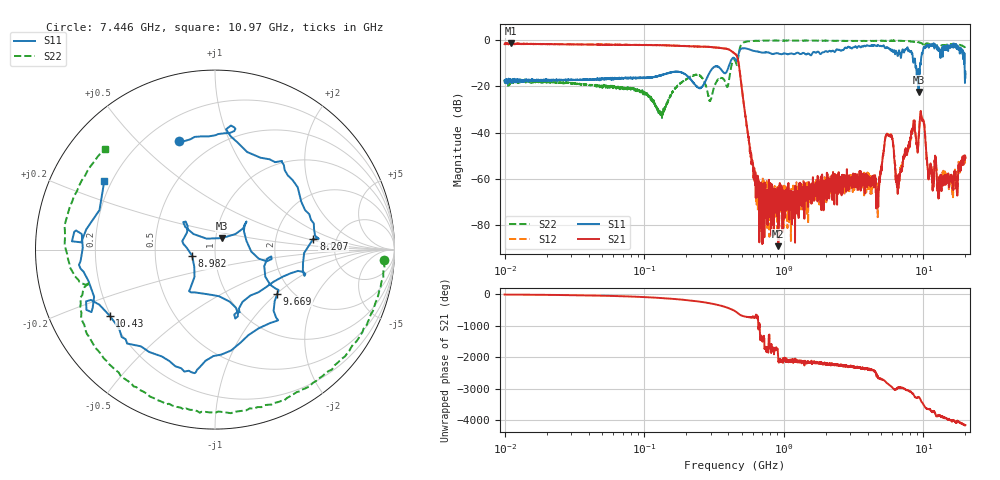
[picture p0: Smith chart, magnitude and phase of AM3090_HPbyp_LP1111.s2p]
# Hz S DB R 50
!freq MagS11 AngS11 MagS21 AngS21 MagS12 AngS12 MagS22 AngS22
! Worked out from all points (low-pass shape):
!   3201 points, 10 MHz to 20 GHz, reference 50 ohm
!   highest |S21| = -1.43 dB at 11.1 MHz (marker M1); lowest = -88.9 dB at 914.2 MHz (marker M2)
!   |S21| within 3 dB of the highest: start of sweep to 413 MHz
!   lowest |S11| = -22.5 dB at 9.242 GHz (marker M3), VSWR 1.16, Z = 53.7 + j6.91 ohm
!   |S11| at or under -10 dB: start of sweep to 410.8 MHz; 8.743 GHz to 9.483 GHz (740 MHz wide, 8.12 % of centre); 19.73 GHz to end of sweep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
!   |S22| runs from -33.7 to -0.2 dB; largest |S21 - S12| = 0.046
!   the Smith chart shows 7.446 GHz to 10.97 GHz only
!   S11 on the Smith chart (normalised r, x): 7.446 GHz: 0.33, +0.67; 8.207 GHz: 3.35, +0.59; 8.982 GHz: 0.77, -0.06; 9.669 GHz: 1.68, -1.01; 10.43 GHz: 0.20, -0.28; 10.97 GHz: 0.17, +0.28
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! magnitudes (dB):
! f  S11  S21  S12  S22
! 10 MHz  -17.5  -1.8  -1.5  -17.7
! 11.1 MHz  -17.4  -1.4  -1.7  -18.7
! 35.55 MHz  -17.2  -2.0  -1.9  -19.1
! 126.1 MHz  -15.6  -2.2  -2.2  -29.8
! 251.7 MHz  -20.8  -2.9  -2.8  -15.6
! 297.9 MHz  -13.4  -3.1  -3.0  -26.2
! 447.2 MHz  -8.2  -5.9  -5.9  -8.8
! 650.9 MHz  -5.0  -63.4  -64.2  -0.4
! 914.2 MHz  -5.9  -88.9  -73.2  -0.3
! 1.59 GHz  -6.1  -63.7  -66.3  -0.2
! 4.708 GHz  -2.2  -68.8  -76.4  -0.4
! 5.639 GHz  -3.7  -41.1  -41.0  -0.3
! 6.534 GHz  -6.8  -64.6  -61.7  -0.3
! 7.446 GHz  -3.9  -47.5  -49.2  -0.5
! 8.207 GHz  -5.2  -39.7  -42.4  -0.7
! 8.982 GHz  -17.6  -45.2  -45.3  -0.9
! 9.242 GHz  -22.5  -41.8  -42.9  -1.0
! 9.669 GHz  -7.4  -32.6  -31.9  -1.3
! 10.43 GHz  -3.2  -45.6  -45.7  -1.6
! 10.97 GHz  -2.8  -59.1  -59.0  -1.6
! 15.92 GHz  -2.5  -61.4  -61.2  -1.8
! 20 GHz  -13.7  -50.9  -49.9  -3.5
